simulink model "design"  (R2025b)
settings: Solver=VariableStepAuto  StartTime=0.0  StopTime=10.0  RelTol=1e-3
InitFcn:
  | SSR=8;
undefined symbols (not defined in the file or in its folder): code, Evaluation, KC705, Kintex, netlist, Platform, xc7k325tffg900
libraries: ModelComposer x4, hlsBasic x2, vmcUtilities x1

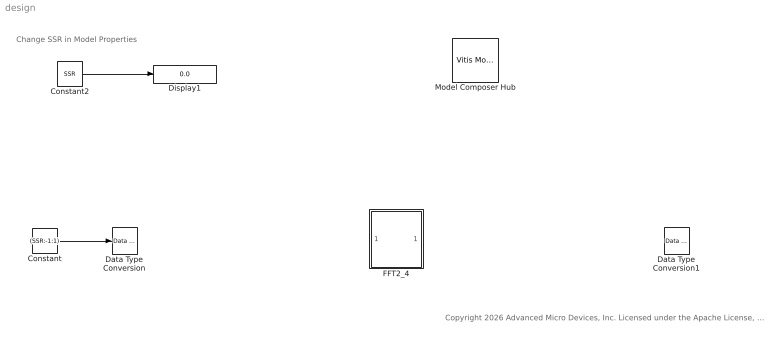
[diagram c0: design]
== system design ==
  note: Change SSR in Model Properties
  note: Copyright 2026 Advanced Micro Devices, Inc. Licensed under the Apache License, Version 2.0 (the "License"); you may not use this file except in compliance with the License. You may obtain a copy of the License at http://www.apache.org/licenses/LICENSE-2.0 Unless required by applicable law or agreed to in writing, software distributed under the License is distributed on an "AS IS" BASIS, WITHOUT WARRANTIES OR CONDITIONS OF ANY KIND, either express or implied. See the License for the specific language governing permissions and limitations under the License.
  Constant : Constant  Value=(SSR:-1:1)  SampleTime=1
  Constant2 : Constant  Value=SSR  VectorParams1D=off  SampleTime=1
  Data Type Conversion : hlsBasic/Data Type Conversion  OutDataType=fixed  TypeExp=''  Signedness=Signed  WordLength=16  FractionalLength=8  RoundingMode=Truncation to minus infinity  OverflowMode=Wrap around
  Data Type Conversion1 : hlsBasic/Data Type Conversion  OutDataType=double  TypeExp=''  Signedness=Signed  WordLength=16  FractionalLength=0  RoundingMode=Truncation to minus infinity  OverflowMode=Wrap around
  Display1 : Display
  FFT2_4 : Subsystem
  Model Composer Hub : vmcUtilities/Vitis Model Composer Hub  Tag=genX  CodeGeneration=off  SubsystemName=Subsystem  StartColumn=1  NumberOfColumns=1  TargetDirectory=./code  exportDesign=off  analyzeDesign=off  validateDesignOnHw=off  ExportType=IP Catalog  IpVendor=xilinx.com  IpLibrary=hls  IpVersion=1.0  IpHWLanguage=Verilog  AieCompilerOptions={}  AieSimulatorOptions={}  CreateTestbench=off  TestbenchStackSize=10  RunRtlSim=off  RunCSim=off  RunAieSim=off  AieSimTimeout=50000  RunAieSimProfiling=off  LaunchVitisAnalyzer=off  PlotOutput=off  RunX86Sim=on  X86SimTimeout=10  GenHwImage=off  GenLibadfXo=off  GenHwValidationCode=off  PlatformType=Not Specified  HwSystemType=Baremetal  HwValidationTarget=hw  ProjDevice=Kintex-7 KC705 Evaluation Platform (xc7k325tffg900-2)  ProjDevicePart=xc7k325tffg900-2  SamplePeriod=-1  ClockFrequency=200  DataPathParallelism=1  xilinxfamily=Kintex7  part=xc7k325t  speed=-3  package=fbg676  directory=./netlist  testbench=off  incr_netlist=off  synthesis_tool=Vivado  clock_wrapper=Clock Enables  dbl_ovrd=According to Block Masks  dcm_input_clock_period=10  sysclk_period=10  simulink_period=1  eval_field=0  LogFileName=''  NThreads=4
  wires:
  Constant/1 -> Data Type Conversion/1
  Data Type Conversion/1 -> ?
  ? -> Data Type Conversion1/1
  FFT2_4/1(O0) -> ?
  FFT2_4/2(O1) -> ?
  ? -> FFT2_4/1(I0)
  ? -> FFT2_4/2(I1)
  Constant2/1 -> Display1/1

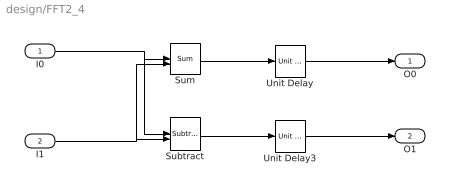
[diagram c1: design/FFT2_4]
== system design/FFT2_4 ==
  I0 : Inport
  I1 : Inport  Port=2
  Subtract : ModelComposer/Subtract
  Sum : ModelComposer/Sum
  Unit Delay : ModelComposer/Unit Delay  InitialCondition=0
  Unit Delay3 : ModelComposer/Unit Delay  InitialCondition=0
  O0 : Outport
  O1 : Outport  Port=2
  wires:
  Sum/1 -> Unit Delay/1
  Unit Delay/1 -> O0/1
  Subtract/1 -> Unit Delay3/1
  Unit Delay3/1 -> O1/1
  I0/1 -> Subtract/1, Sum/1
  I1/1 -> Subtract/2, Sum/2
